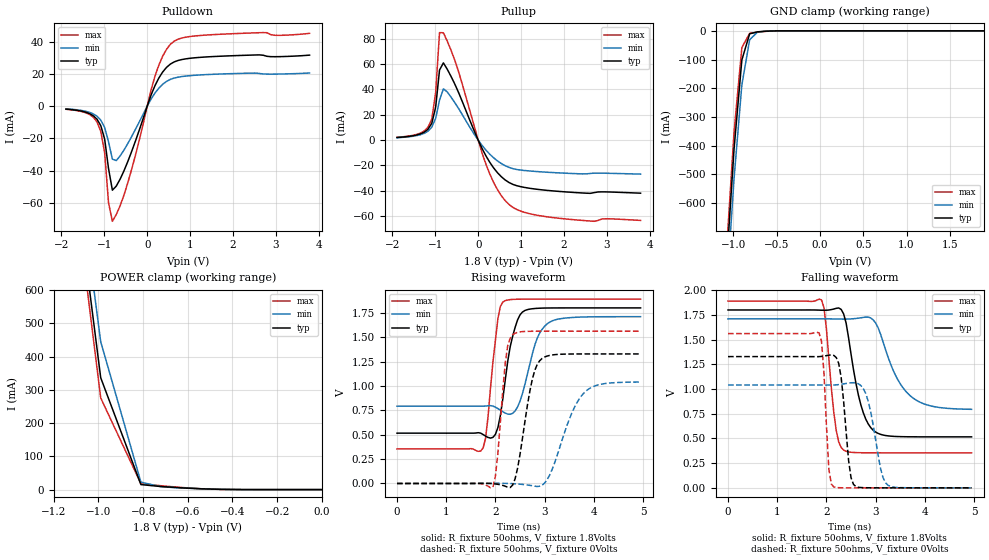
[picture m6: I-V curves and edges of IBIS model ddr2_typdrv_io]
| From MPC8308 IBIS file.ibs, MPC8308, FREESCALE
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[Model]   ddr2_typdrv_io   |
Model_type   I/O
Vinl = 0.87
Vinh = 0.93
Vmeas = 0.9
Cref = 1E-11
Rref = 50
Vref = 0.9
| variable   typ   min   max
C_comp   1.17p   1.10p   1.23p
[Model Spec]
| subparameter   typ   min   max
S_overshoot_high  3.300   3.135   3.465
S_overshoot_low   -200.00m  -100.00m  -300.00m
D_overshoot_high  4.000   4.000   4.000
D_overshoot_low   -1.000   -1.000   -1.000
D_overshoot_time  1.000n   1.000n   1.000n
| variable   typ   min   max
[Temperature Range]   25.0   -40.0   125.0
| variable   typ   min   max
[Pullup Reference]   1.800V   1.710V   1.890V
| variable   typ   min   max
[Pulldown Reference]   0.000V   0.000V   0.000V
| variable   typ   min   max
[POWER_Clamp_Reference]   1.800V   1.710V   1.890V
| variable   typ   min   max
[GND_Clamp_Reference]   0.000V   0.000V   0.000V
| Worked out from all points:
|   slope of the pulldown table from 0 to 0.27 V, typ, clamps not added: 15.5 ohm
|   slope of the pullup table from 0 to 0.27 V, typ, clamps not added: 15.4 ohm
|   GND clamp passes 1 mA (typ) near -0.59 V on its own axis
|   POWER clamp passes 1 mA (typ) near -0.47 V on its own axis
|   rising waveform, R_fixture 50ohms, V_fixture 1.8Volts: 20-80 % time 246ps typ, 306ps min, 181ps max; typ from 0.516 V to 1.8 V
|   rising waveform, R_fixture 50ohms, V_fixture 0Volts: 20-80 % time 259ps typ, 461ps min, 153ps max; typ from 0 V to 1.33 V
|   falling waveform, R_fixture 50ohms, V_fixture 1.8Volts: 20-80 % time 299ps typ, 494ps min, 173ps max; typ from 1.8 V to 0.516 V
|   falling waveform, R_fixture 50ohms, V_fixture 0Volts: 20-80 % time 143ps typ, 226ps min, 99.1ps max; typ from 1.33 V to 0 V
[Pulldown]
| pulldown in the table = pulldown subtract gnd_clamp
|Voltage   I(typ)   I(min)   I(max)
-1.89V    -1.814mA   -1.621mA   -1.914mA
-1.17V    -8.014mA   -6.166mA   -9.649mA
-1.08V    -12.08mA   -8.646mA   -15.64mA
-990mV    -20.44mA   -13.21mA   -28.88mA
-900mV    -38.7mA    -22.11mA   -59.93mA
-810mV    -52.14mA   -32.89mA   -71.45mA
-720mV    -49.61mA   -33.72mA   -67.26mA
-450mV    -34.25mA   -23.11mA   -47.41mA
180mV     12.68mA    8.129mA    18.5mA
540mV     26.16mA    16.66mA    38.43mA
1.26V     30.38mA    19.46mA    43.95mA
3.78V     31.7mA     20.61mA    45.23mA
[Pullup]
| pullup in the table = pullup subtract power_clamp
|Voltage   I(typ)   I(min)   I(max)
-1.89V    2.087mA    1.909mA    2.263mA
-1.35V    4.875mA    4.247mA    5.499mA
-1.08V    13.33mA    10.25mA    16.64mA
-990mV    26.04mA    17.18mA    37.68mA
-900mV    55.36mA    31.66mA    84.9mA
-810mV    60.98mA    40.51mA    84.73mA
-450mV    37.05mA    24.61mA    53.31mA
180mV     -12.39mA   -7.822mA   -18.96mA
450mV     -25.74mA   -16.42mA   -39.15mA
720mV     -33.48mA   -21.53mA   -50.84mA
1.71V     -39.96mA   -25.52mA   -60.96mA
3.78V     -41.85mA   -26.8mA    -63.34mA
[GND_clamp]
|Voltage   I(typ)   I(min)   I(max)
-1.89V    -5.289A    -5.314A    -5.291A
-1.08V    -830.5mA   -924.5mA   -780.6mA
-990mV    -411.5mA   -514.7mA   -352.7mA
-900mV    -101.5mA   -188.4mA   -58.29mA
-810mV    -10.46mA   -31.1mA    -8.864mA
-720mV    -3.532mA   -4.591mA   -4.66mA
-630mV    -1.451mA   -1.339mA   -1.97mA
1.89V     11.74nA    4.438uA    11.9pA
[POWER_clamp]
|Voltage   I(typ)   I(min)   I(max)
-1.71V    4.942A     4.957A     4.954A
-1.08V    811.3mA    908.1mA    762.8mA
-990mV    336.3mA    444.6mA    275.5mA
-810mV    15.09mA    22.51mA    17.99mA
-720mV    9.216mA    8.568mA    11.65mA
-630mV    5.341mA    4.938mA    6.448mA
-450mV    673.8uA    1mA        542.4uA
0V        210.7pA    7.657nA    11.9pA
[Ramp]
|Voltage   I(typ)   I(min)   I(max)
dV/dt_f   0.78/301.271p 0.56/500.394p 0.93/172.921p
dV/dt_r   0.82/265.759p 0.64/472.089p 0.97/157.686p
R_load=50ohms
| R_load was connected to ground for Ramp_up test and power for Ramp_dn test
[Rising_Waveform]
R_fixture=50ohms
V_fixture=1.8Volts
V_fixture_min=1.71Volts
V_fixture_max=1.89Volts
|C_fixture=1E-15f
|L_fixture=1E-15h
|C_dut=1E-15fh
|R_dut=0.001ohm
|L_dut=1E-12h
|time   V(typ)   V(min)   V(max)
0s        515.9mV    792.4mV    354.5mV
1.75ns    501.7mV    792.6mV    364mV
1.85ns    472mV      796.9mV    683mV
2ns       503.7mV    782.5mV    1.467V
2.15ns    867mV      735.8mV    1.859V
2.3ns     1.401V     709.6mV    1.885V
2.55ns    1.758V     922.6mV    1.89V
2.85ns    1.796V     1.49V      1.89V
3.1ns     1.799V     1.653V     1.89V
4.95ns    1.8V       1.71V      1.89V
[Rising_Waveform]
R_fixture=50ohms
V_fixture=0Volts
|C_fixture=1E-15f
|L_fixture=1E-15h
|C_dut=1E-15fh
|R_dut=0.001ohm
|L_dut=1E-12h
|time   V(typ)   V(min)   V(max)
0s        7.153nV    673.7nV    82.59pV
1.95ns    -2.101mV   1.885mV    -38.29mV
2.05ns    -8.48mV    1.995mV    310.5mV
2.25ns    -38.8mV    603.1uV    1.412V
2.4ns     48.32mV    -3.169mV   1.54V
2.75ns    1.069V     -23.29mV   1.561V
2.9ns     1.259V     -28.2mV    1.561V
3.1ns     1.313V     83.95mV    1.561V
3.8ns     1.328V     928.3mV    1.561V
4.95ns    1.328V     1.04V      1.561V
[Falling_Waveform]
R_fixture=50ohms
V_fixture=1.8Volts
V_fixture_min=1.71Volts
V_fixture_max=1.89Volts
|C_fixture=1E-15f
|L_fixture=1E-15h
|C_dut=1E-15fh
|R_dut=0.001ohm
|L_dut=1E-12h
|time   V(typ)   V(min)   V(max)
0s        1.8V       1.71V      1.89V
1.9ns     1.798V     1.71V      1.902V
2ns       1.798V     1.71V      1.61V
2.2ns     1.817V     1.709V     578.9mV
2.35ns    1.76V      1.708V     382.3mV
2.7ns     839.4mV    1.721V     355.5mV
2.95ns    583.5mV    1.7V       354.6mV
3.4ns     520.3mV    1.143V     354.5mV
3.7ns     516.8mV    933.6mV    354.5mV
4.95ns    515.9mV    794.8mV    354.5mV
[Falling_Waveform]
R_fixture=50ohms
V_fixture=0Volts
|C_fixture=1E-15f
|L_fixture=1E-15h
|C_dut=1E-15fh
|R_dut=0.001ohm
|L_dut=1E-12h
|time   V(typ)   V(min)   V(max)
0s        1.328V     1.041V     1.561V
1.85ns    1.328V     1.041V     1.568V
1.95ns    1.334V     1.04V      1.164V
2.05ns    1.343V     1.04V      185.5mV
2.15ns    1.34V      1.041V     9.785mV
2.3ns     1.116V     1.048V     976.7uV
2.55ns    35.15mV    1.064V     83.81uV
2.8ns     1.352mV    953.2mV    7.48uV
3.25ns    80.77uV    27mV       -106.9nV
4.95ns    2.783nV    9.64uV     -13.88nV
